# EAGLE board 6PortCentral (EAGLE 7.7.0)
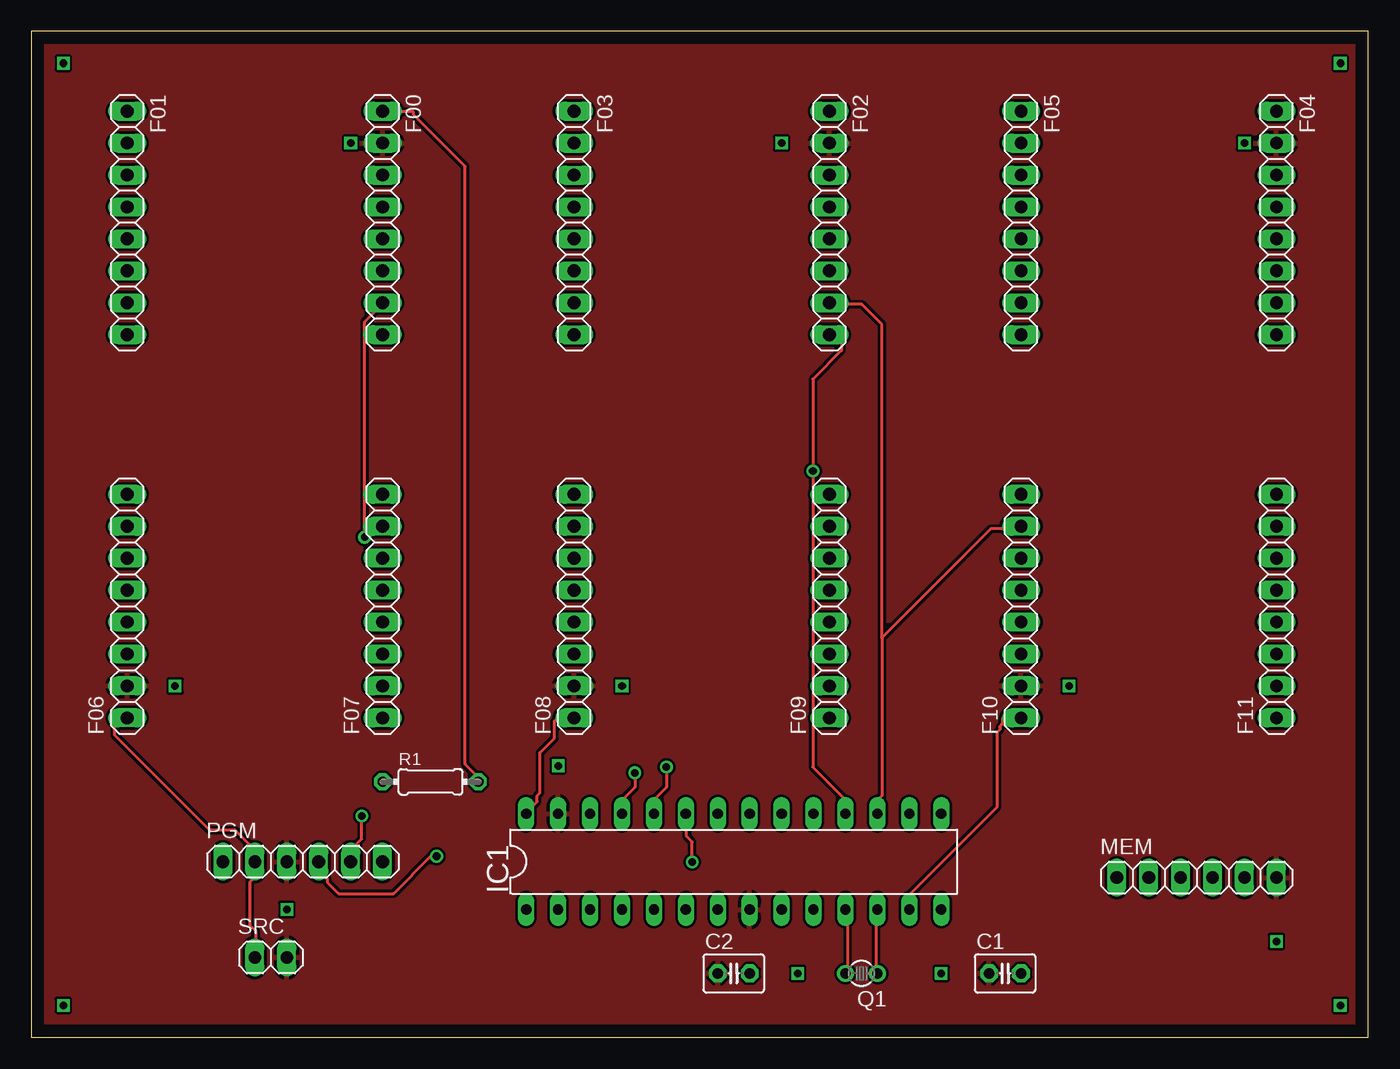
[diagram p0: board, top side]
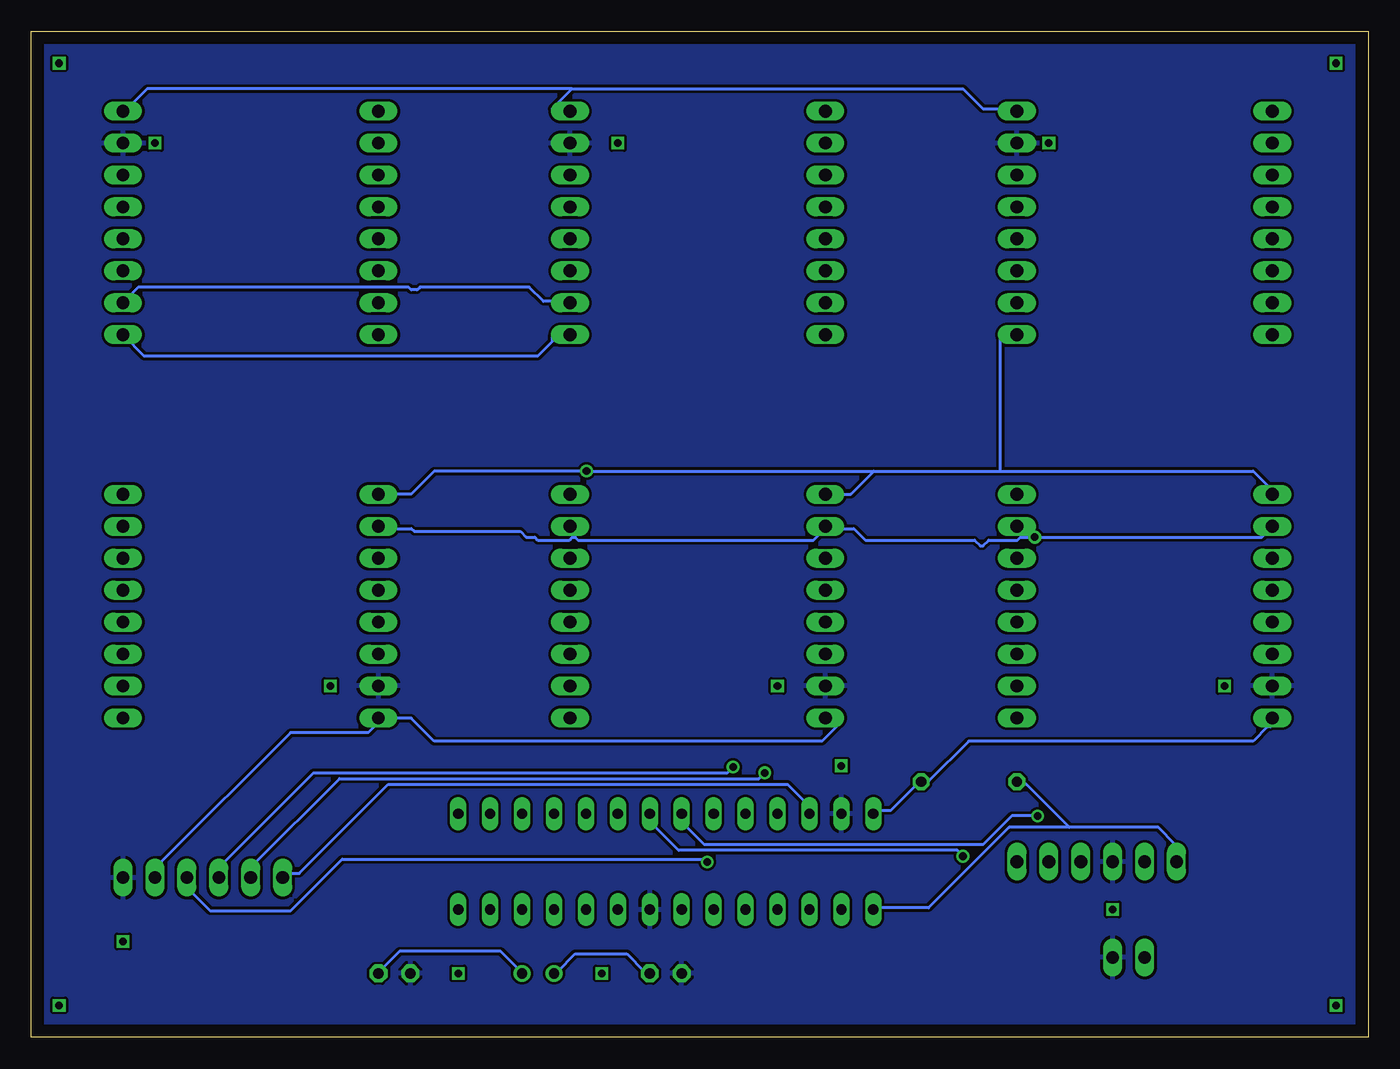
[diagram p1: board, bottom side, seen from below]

Size 106.35 x 80 mm. Coordinates in mm from the lower left corner, seen from the top.
Outline: 0,0 106.35,0 106.35,80 0,80 0,0
Copper layers (1*16): Top 0.035mm / dielectric 1.5mm / Bottom 0.035mm
Design rules "default": minimum track width 10mil, minimum drill 24mil, track to track 8mil, track to pad 8mil, pad to pad 8mil, via to via 8mil, smd to smd 8mil, copper to edge 40mil, drill to drill 8mil, minimum pad ring 10mil, minimum via ring 8mil, stop-mask expansion 4mil, vias tented up to drill 0mil, thermal gap 10mil

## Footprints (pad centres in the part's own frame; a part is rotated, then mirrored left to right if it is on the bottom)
C025-030X050 = drill 0.813 pad 1.422 octagon: 1 -1.27,0; 2 1.27,0
1X08 = drill 1.016 long: 1 -8.89,0; 2 -6.35,0; 3 -3.81,0; 4 -1.27,0; 5 1.27,0; 6 3.81,0; 7 6.35,0; 8 8.89,0
DIL28-3 = drill 0.813 long: 1 -16.51,-3.81; 2 -13.97,-3.81; 3 -11.43,-3.81; 4 -8.89,-3.81; 5 -6.35,-3.81; 6 -3.81,-3.81; 7 -1.27,-3.81; 8 1.27,-3.81; 9 3.81,-3.81; 10 6.35,-3.81; 11 8.89,-3.81; 12 11.43,-3.81; 13 13.97,-3.81; 14 16.51,-3.81; 15 16.51,3.81; 16 13.97,3.81; 17 11.43,3.81; 18 8.89,3.81; 19 6.35,3.81; 20 3.81,3.81; 21 1.27,3.81; 22 -1.27,3.81; 23 -3.81,3.81; 24 -6.35,3.81; 25 -8.89,3.81; 26 -11.43,3.81; 27 -13.97,3.81; 28 -16.51,3.81
1X06 = drill 1.016 long: 1 -6.35,0; 2 -3.81,0; 3 -1.27,0; 4 1.27,0; 5 3.81,0; 6 6.35,0
TC26V = drill 0.813: 1 -1.27,0; 2 1.27,0
0204/7 = drill 0.813 octagon: 1 -3.81,0; 2 3.81,0
1X02 = drill 1.016 long: 1 -1.27,0; 2 1.27,0

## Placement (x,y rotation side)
C1  [C025-030X050]  77.47,5.08 0 top
C2  [C025-030X050]  55.88,5.08 0 top
F00  [1X08]  27.94,64.77 270 top
F01  [1X08]  7.62,64.77 270 top
F02  [1X08]  63.5,64.77 270 top
F03  [1X08]  43.18,64.77 270 top
F04  [1X08]  99.06,64.77 270 top
F05  [1X08]  78.74,64.77 270 top
F06  [1X08]  7.62,34.29 90 top
F07  [1X08]  27.94,34.29 90 top
F08  [1X08]  43.18,34.29 90 top
F09  [1X08]  63.5,34.29 90 top
F10  [1X08]  78.74,34.29 90 top
F11  [1X08]  99.06,34.29 90 top
IC1  PIC24FJ64GA002  [DIL28-3]  55.88,13.97 0 top
MEM  [1X06]  92.71,12.7 0 top
PGM  [1X06]  21.59,13.97 0 top
Q1  [TC26V]  66.04,5.08 180 top
R1  10k  [0204/7]  31.75,20.32 0 top
SRC  [1X02]  19.05,6.35 0 top

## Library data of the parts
C1 C2 = adafruit
F00 F01-F09 F10 F11 MEM PGM SRC = pinhead
IC1 = microchip; MPN: PIC24FJ64GA002-I/SP; OC_FARNELL: 1332298; OC_NEWARK: 88K6132
Q1 = crystal; OC_FARNELL: unknown; OC_NEWARK: unknown
R1 = resistor

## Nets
GND: C1.1 C2.1 F00.2 F02.2 F04.2 F06.2 F08.2 F10.2 IC1.8 IC1.27 MEM.6 PGM.3 SRC.2
MISO: IC1.23 MEM.4
MOSI: IC1.24 MEM.3
N$1: IC1.1 PGM.1 R1.1
N$2: C1.2 IC1.12 Q1.1
N$3: C2.2 IC1.11 Q1.2
N$4: IC1.21 PGM.4
N$5: IC1.22 PGM.5
SCL: F00.7 F02.7 F04.7 F06.7 F08.7 F10.7 IC1.17
SDA: F00.8 F02.8 F04.8 F06.8 F08.8 F10.8 IC1.18
SPICK: IC1.25 MEM.2
SS: IC1.26 MEM.1
VDD: F00.1 F02.1 F04.1 F06.1 F08.1 F10.1 IC1.13 IC1.28 MEM.5 PGM.2 R1.2 SRC.1
VDDCORE: IC1.20

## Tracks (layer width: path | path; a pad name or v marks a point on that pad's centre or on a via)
GND
  pour Bottom: -1.27,81.28 107.95,81.28 107.95,-1.27 -1.27,-1.27
  pour Top: -1.27,81.28 107.95,81.28 107.95,-1.27 -1.27,-1.27
MISO  (via drill 0.61)
  Top 0.254: v52.58,13.95 52.58,15.54 52.12,16 52.12,17.6 IC1.23
  Bottom 0.254: v52.58,13.95 52.81,14.17 81.61,14.17 85.72,10.06 92.13,10.06 93.95,11.89 93.95,12.57 MEM.4
MOSI  (via drill 0.61)
  Top 0.254: v50.52,21.49 50.52,19.89 49.61,18.97 49.61,17.83 IC1.24
  Bottom 0.254: v50.52,21.49 50.98,21.03 83.9,21.03 91.44,13.49 MEM.3
N$1
  Bottom 0.254: 23.77,16.69 27.2,20.12 27.89,20.12 R1.1 | 23.77,16.69 16.69,16.69 15.32,15.32 15.32,14.17 PGM.1 | 23.77,16.69 28.57,16.69 34.98,10.29 39.32,10.29 IC1.1
N$2
  Top 0.254: Q1.1 67.21,5.26 67.21,10.06 IC1.12
  Bottom 0.254: C1.2 78.64,5.26 77.04,6.86 69.04,6.86 67.67,5.49 67.67,5.26 67.44,5.26 Q1.1
N$3
  Top 0.254: Q1.2 64.92,5.26 64.92,10.06 IC1.11
  Bottom 0.254: C2.2 57.15,5.26 57.61,5.26 58.98,6.63 63.09,6.63 64.47,5.26 64.69,5.26 Q1.2
N$4  (via drill 0.61)
  Top 0.254: v32.23,14.4 31.77,14.4 28.8,11.43 24.46,11.43 23.55,12.34 23.55,12.57 22.86,13.26 PGM.4
  Bottom 0.254: v32.23,14.4 32.69,14.86 54.86,14.86 56.69,16.69 56.69,17.14 57.15,17.6 IC1.21
N$5  (via drill 0.61)
  Top 0.254: v26.29,17.6 26.29,15.77 25.6,15.09 25.6,14.17 PGM.5
  Bottom 0.254: v26.29,17.6 28.35,17.6 30.63,15.32 52.81,15.32 54.18,16.69 54.41,16.69 54.41,17.6 IC1.22
N$6  (via drill 0.6)
  other vias: 2.54,77.47
N$7  (via drill 0.6)
  other vias: 104.14,77.47
N$8  (via drill 0.6)
  other vias: 104.14,2.54
N$9  (via drill 0.6)
  other vias: 2.54,2.54
N$10  (via drill 0.6)
  other vias: 20.32,10.16
N$11  (via drill 0.6)
  other vias: 11.43,27.94
N$12  (via drill 0.6)
  other vias: 46.99,27.94
N$13  (via drill 0.6)
  other vias: 82.55,27.94
N$14  (via drill 0.6)
  other vias: 99.06,7.62
N$15  (via drill 0.6)
  other vias: 72.39,5.08
N$16  (via drill 0.6)
  other vias: 60.96,5.08
N$17  (via drill 0.6)
  other vias: 41.91,21.59
N$18  (via drill 0.6)
  other vias: 25.4,71.12
N$19  (via drill 0.6)
  other vias: 59.69,71.12
N$20  (via drill 0.6)
  other vias: 96.52,71.12
SCL  (via drill 0.61)
  Top 0.254: v26.52,39.78 26.52,56.92 27.89,58.29 29.03,58.29 F00.7 | 67.67,31.77 67.67,19.2 67.44,18.97 67.44,17.83 IC1.17 | 67.67,31.77 76.35,40.46 77.27,40.46 F10.7 | 67.67,31.77 67.67,56.69 66.06,58.29 64.92,58.29 F02.7
  Bottom 0.254: F06.7 6.4,40.46 7.77,40.46 8.46,39.78 v26.52,39.78 27.66,39.78 27.89,39.55 30.18,39.55 30.63,39.09 30.86,39.09 31.32,39.55 40.01,39.55 40.92,40.46 41.83,40.46 F08.7 42.06,40.46 43.2,40.46 44.12,39.55 62.87,39.55 63.09,39.78 63.32,39.78 63.55,39.55 66.06,39.55 66.29,39.78 66.98,39.78 67.44,40.23 75.89,40.23 76.12,40.46 77.27,40.46 F10.7 | F04.7 100.13,58.52 98.98,58.52 97.84,59.66 76.35,59.66 76.12,59.44 75.67,59.44 75.44,59.66 66.75,59.66 65.61,58.52 64.92,58.52 F02.7
SDA  (via drill 0.61)
  Top 0.254: IC1.18 64.69,17.83 64.69,18.97 62.18,21.49 v62.18,45.03 62.18,52.35 64.47,54.63 64.47,55.55 64.69,55.78 F02.8
  Bottom 0.254: 39.32,45.03 29.26,45.03 | 29.26,45.03 9.14,45.03 7.54,43.43 6.63,43.43 6.4,43.2 F06.8 | 39.32,45.03 41.15,43.2 41.83,43.2 F08.8 | 29.26,45.03 29.26,55.78 F00.8 | F10.8 77.27,43.2 76.12,43.2 74.3,45.03 v62.18,45.03 39.32,45.03 | F04.8 100.13,55.78 98.98,55.78 97.38,54.18 66.06,54.18 64.92,55.32 64.92,55.78 F02.8
SPICK  (via drill 0.61)
  Top 0.254: v48.01,21.03 48.01,19.89 47.09,18.97 47.09,17.83 IC1.25
  Bottom 0.254: v48.01,21.03 48.46,20.57 81.84,20.57 88.7,13.72 88.7,12.8 MEM.2
SS
  Bottom 0.254: IC1.26 44.58,17.83 44.58,18.75 44.81,18.75 46.18,20.12 77.95,20.12 85.04,13.03 85.95,13.03 86.18,12.8 MEM.1
VDD
  Top 0.254: IC1.13 69.95,10.29 69.95,11.43 76.81,18.29 76.81,24.23 77.04,24.46 77.04,24.69 77.27,24.92 77.27,25.38 F10.1 | F08.1 41.83,25.38 41.6,25.15 41.6,23.77 40.46,22.63 40.46,19.43 40.23,19.2 40.23,18.75 39.55,18.06 39.55,17.83 IC1.28 | SRC.1 17.83,6.4 17.83,8.46 17.37,8.91 17.37,12.34 17.6,12.57 17.6,13.95 PGM.2 17.6,14.17 17.6,15.09 16.23,16.46 14.17,16.46 6.63,24 6.63,25.15 6.4,25.38 F06.1 | F00.1 29.26,73.61 30.4,73.61 30.4,73.38 34.52,69.27 34.52,21.72 35.43,20.8 35.43,20.34 R1.2
  Bottom 0.254: 63.32,75.44 32.23,75.44 30.63,73.84 29.26,73.84 F00.1 | 63.32,75.44 64.92,73.84 F02.1 | 63.32,75.44 97.16,75.44 98.53,74.07 98.75,74.07 98.98,73.84 100.13,73.84 F04.1 | MEM.5 96.47,12.8 96.01,13.26 96.01,13.95 85.72,24.23 79.55,24.23 78.41,25.38 77.5,25.38 F10.1 77.27,25.38 76.12,25.38 74.3,23.55 43.43,23.55 42.06,24.92 42.06,25.38 F08.1 | IC1.28 39.09,18.06 37.95,18.06 35.89,20.12 35.66,20.12 R1.2 35.43,20.34 34.98,20.34 31.77,23.55 9.14,23.55 8,24.69 7.77,24.69 7.09,25.38 6.4,25.38 F06.1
